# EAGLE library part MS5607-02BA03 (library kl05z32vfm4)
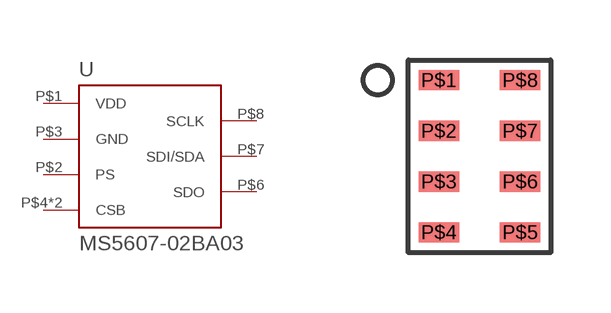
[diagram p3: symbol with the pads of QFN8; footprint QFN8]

Designator prefix -

## MS5607-02BA03  [QFN8]
P$1  VDD
P$2  PS
P$3  GND
P$4  CSB
P$5  CSB
P$6  SDO
P$7  SDI/SDA
P$8  SCLK

## Footprint QFN8 (pad centres in mm)
smd 1.016 x 0.508: P$1 -1.27,1.27; P$2 -1.27,0; P$3 -1.27,-1.27; P$4 -1.27,-2.54; P$5 0.762,-2.54; P$6 0.762,-1.27; P$7 0.762,0; P$8 0.762,1.27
